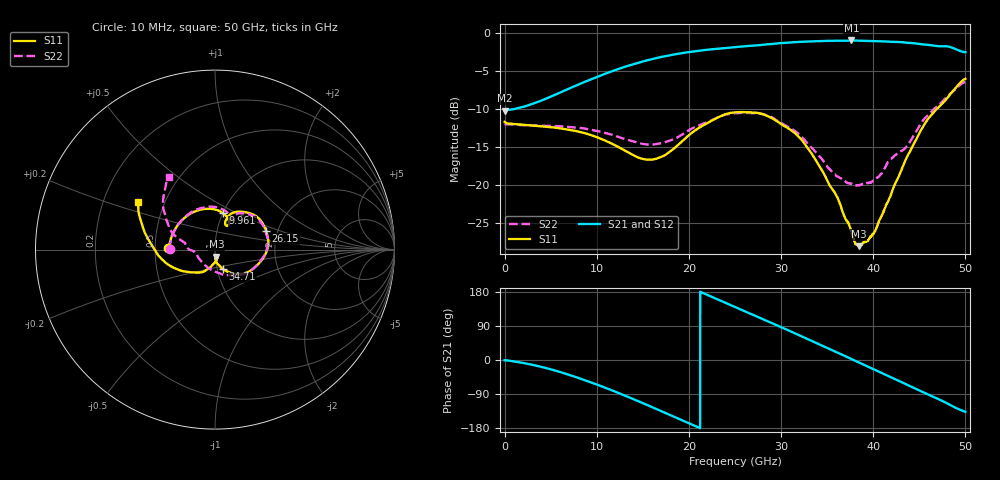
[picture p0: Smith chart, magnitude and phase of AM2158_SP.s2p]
!Keysight Technologies,N5245B,MY58422270,A.16.20.02
!Date: Thursday, March 12, 2026 19:32:28
!Correction: S11(C  2-Port  )
!S21(C  2-Port  )
!S12(C  2-Port  )
!S22(C  2-Port  )
!S2P File: Measurements: S11, S21, S12, S22:
# Hz S  dB  R 50
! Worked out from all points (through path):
!   6401 points, 10 MHz to 50 GHz, reference 50 ohm
!   highest |S21| = -0.93 dB at 37.64 GHz (marker M1); lowest = -10.2 dB at 10 MHz (marker M2)
!   group delay of S21, straight-line fit = 28.8 ps
!   lowest |S11| = -28.0 dB at 38.42 GHz (marker M3), VSWR 1.08, Z = 50.6 - j3.97 ohm
!   |S11| at or under -10 dB: start of sweep to 46.84 GHz
!   |S22| runs from -20.0 to -6.4 dB; largest |S21 - S12| = 0.0053
!   S11 on the Smith chart (normalised r, x): 10 MHz: 0.59, +0.01; 9.961 GHz: 1.00, +0.43; 26.15 GHz: 1.74, +0.40; 34.71 GHz: 1.06, -0.24; 50 GHz: 0.35, +0.25
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1e7  -11.64 177.9  -10.16 -0.6  -10.15 -0.5  -11.96 179.2
4.415369e9  -12.26 127.8  -8.63 -20.7  -8.63 -20.7  -12.15 127.7
8.34427e9  -13.00 90.1  -6.56 -50.0  -6.56 -50.0  -12.45 91.5
9.961134e9  -13.63 77.7  -5.76 -64.2  -5.76 -64.2  -12.81 79.8
1.360884e10  -15.78 61.2  -4.19 -99.5  -4.19 -99.4  -14.09 62.8
1.667854e10  -16.40 67.6  -3.19 -131.3  -3.19 -131.3  -14.51 62.0
1.892809e10  -14.58 69.2  -2.66 -155.4  -2.66 -155.4  -13.56 61.1
2.104485e10  -12.47 61.5  -2.29 -178.0  -2.29 -177.9  -12.13 55.3
2.295072e10  -11.18 47.9  -2.04 161.6  -2.04 161.6  -11.15 44.5
2.5005e10  -10.39 31.0  -1.81 139.9  -1.81 140.0  -10.50 30.3
2.61454e10  -10.37 20.1  -1.69 127.9  -1.69 127.9  -10.46 21.1
2.987121e10  -11.79 -17.2  -1.29 88.2  -1.30 88.2  -11.65 -14.2
3.333927e10  -15.86 -54.3  -1.05 50.2  -1.04 50.2  -15.05 -54.3
3.4714e10  -18.60 -68.3  -1.00 35.0  -1.00 35.1  -17.02 -75.1
3.76431e10  -26.12 -89.4  -0.93 2.5  -0.94 2.6  -19.78 -128.8
3.842419e10  -27.99 -79.1  -0.96 -6.3  -0.96 -6.3  -19.98 -145.1
4.004105e10  -26.36 -75.0  -1.02 -24.3  -1.01 -24.2  -19.35 -168.0
4.167354e10  -21.94 -96.3  -1.09 -42.4  -1.08 -42.3  -16.82 179.7
4.372001e10  -16.11 -125.0  -1.23 -65.8  -1.23 -65.7  -14.75 166.1
4.572742e10  -11.62 -159.1  -1.49 -88.3  -1.48 -88.2  -11.01 154.4
4.786761e10  -8.75 173.4  -1.70 -112.5  -1.69 -112.3  -8.49 140.4
5e10  -5.98 148.3  -2.48 -136.6  -2.52 -136.3  -6.38 122.6
